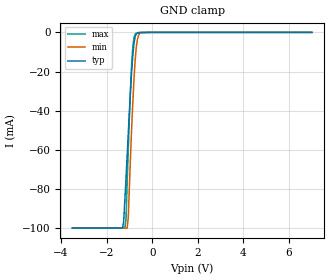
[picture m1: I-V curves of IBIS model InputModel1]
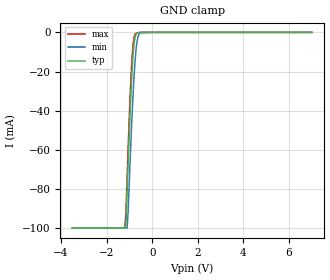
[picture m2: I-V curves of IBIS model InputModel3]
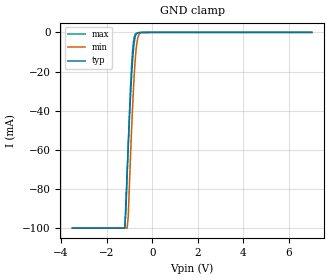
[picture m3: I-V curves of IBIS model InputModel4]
[IBIS Ver]   2.1
[File name]   e_032sa3.ibs   | e_= TSOP, f032sa= abbr chip name, 3= 3.3V Vcc
[File Rev]   2.00
[Date]   26-February-96
[Source]   File generated from lab measurements at Intel Corporation
[Notes]   Rev 2.00   All data from actual measurements performed in a lab.
[Disclaimer] INTEL DEVELOPER'S SOFTWARE LICENSE AGREEMENT
| BY USING THIS SOFTWARE, YOU ARE AGREEING TO BE BOUND
| BY THE TERMS OF THIS AGREEMENT.  DO NOT USE THE SOFTWARE
| UNTIL YOU HAVE CAREFULLY READ AND AGREED TO THE FOLLOWING
| TERMS AND CONDITIONS.  IF YOU DO NOT AGREE TO THE TERMS
| OF THIS AGREEMENT, PROMPTLY RETURN THE SOFTWARE PACKAGE
| AND ANY ACCOMPANYING ITEMS.
| IF YOU USE THIS SOFTWARE, YOU WILL BE BOUND BY THE TERMS
| OF THIS AGREEMENT
| LICENSE: Intel Corporation ("Intel") grants you the non-exclusive right
| to use the enclosed software program ("Software").  You will not use,
| copy, modify, rent, sell or transfer the Software or any portion
| thereof, except as provided in this Agreement.
| System OEM Developers may:
| 1.   Copy the Software for support, backup or archival purposes;
| 2.   Install, use, or distribute Intel owned Software in object code
|   only;
| 3.   Modify and/or use Software source code that Intel directly makes
|   available to you as an OEM Developer;
| 4.   Install, use, modify, distribute, and/or make or have made
|   derivatives ("Derivatives") of Intel owned Software under the
|   terms and conditions in this Agreement, ONLY if you are a System
|   OEM Developer and NOT an end-user.
| RESTRICTIONS:
| YOU WILL NOT:
| 1.   Copy the Software, in whole or in part, except as provided for
|   in this Agreement;
| 2.   Decompile or reverse engineer any Software provided in object
|   code format;
| 3.   Distribute any Software or Derivative code to any end-users,
|   unless approved by Intel in a prior writing.
| TRANSFER: You may transfer the Software to another OEM
| Developer if thereceiving party agrees to the terms of this
| Agreement at the sole risk of any receiving party.
| OWNERSHIP AND COPYRIGHT OF SOFTWARE:
| Title to the Software and all copies thereof remain with Intel
| or its vendors.  The Software iscopyrighted and is protected by
| United States and international copyright laws.  You will not
| remove the copyright notice from the Software.  You agree to
| prevent any unauthorized copying of the Software.
| DERIVATIVE WORK: OEM Developers that make or have made
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[Copyright]   Copyright 1996, Intel Corporation, All Rights Reserved
[Component]   E28F032SA   | 56-lead TSOP package, 28F032SA
[Manufacturer]  Intel   | FlashFile(tm) Memory
|   | operating in 3.3 V Vcc range
|********************Pin and Package Definitions*********************
[Package]
|The following values apply for the Copper leadframe.
|Variable   typ   min   max
R_pkg   48m   41m   54m
L_pkg   4.92nH   4.44nH   5.39nH
C_pkg   0.48pF   0.45pF   0.50pF
|The following values apply for the Alloy-42 leadframe.
|Variable   typ   min   max
|R_pkg   195m   180m   210m
|L_pkg   4.92nH   4.44nH   5.39nH
|C_pkg   0.48pF   0.45pF   0.50pF
|***********************Pin Defintions*************************************
[Pin] signal_name   model_name   R_pin   L_pin   C_pin
  1   3/5#   InputModel1
  2   CE1#   InputModel5
  3   CE2#   InputModel6
  4   A20   InputModel3
  5   A19   InputModel3
  6   A18   InputModel1
  7   A17   InputModel1
  8   A16   InputModel1
  9   VCC   POWER
 10   A15   InputModel1
 11   A14   InputModel3
 12   A13   InputModel1
 13   A12   InputModel1
 14   CE0#   InputModel1
 15   VPP   POWER
 16   RP#   InputModel4
 17   A11   InputModel1
 18   A10   InputModel1
 19   A9   InputModel1
 20   A8   InputModel1
 21   GND   GND
 22   A7   InputModel1
 23   A6   InputModel1
 24   A5   InputModel1
 25   A4   InputModel1
 26   A3   InputModel1
 27   A2   InputModel1
 28   A1   InputModel1
 29   NC   InputModel2
 30   NC   InputModel2
 31   BYTE#   InputModel1
 32   A0   InputModel1
 33   DQ0   InputOutput
 34   DQ8   InputOutput
 35   DQ1   InputOutput
 36   DQ9   InputOutput
 37   VCC   POWER
 38   DQ2   InputOutput
 39   DQ10   InputOutput
 40   DQ3   InputOutput
 41   DQ11   InputOutput
 42   GND   GND
 43   VCC   POWER
 44   DQ4   InputOutput
 45   DQ12   InputOutput
 46   DQ5   InputOutput
 47   DQ13   InputOutput
 48   GND   GND
 49   DQ6   InputOutput
 50   DQ14   InputOutput
 51   DQ7   InputOutput
 52   DQ15   InputOutput
 53   RY/BY#   OpenDrainOutput
 54   OE#   InputModel1
 55   WE#   InputModel4
 56   WP#   InputModel1
|*************************Input Model 2***************************
[Model]   InputModel2
Model_type   Input
|   For NC (Pins 29 & 30)
Vinl = 0.8V
Vinh = 2.0V
| Variable   typ   min   max
C_comp   5.61p   NA   7.6p
[Voltage Range]   3.3V   3.0V   3.6V
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| Models and submodels in the file (8): InputModel1 (Input), InputModel2 (Input), InputModel3 (Input), InputModel4 (Input), InputModel5 (Input), InputModel6 (Input), InputOutput (I/O), OpenDrainOutput (Open_drain)
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|**********************Input Model 1 *******************************
[Model]   InputModel1
Model_type   Input
|   For pin1(3/5#), CE0#, OE#, WP#, BYTE#, A[18:15], A[13:0]
Vinl = 0.8V
Vinh = 2.0V
|Variable   typ   min   max
C_comp   5.61p   NA   7.6p
[Voltage Range]   3.3V   3.0V   3.6V
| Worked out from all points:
|   GND clamp passes 1 mA (typ) near -0.71 V on its own axis
[GND_clamp]
|Voltage I(typ)   I(min)   I(max)
-3.5V     -100mA     -100mA     -100mA
-1.3V     -100mA     -100mA     -100mA
-1.25V    -96.28mA   -100mA     -100mA
-1.2V     -85.5mA    -100mA     -100mA
-1.15V    -74.82mA   -100mA     -95.38mA
-1.1V     -63.19mA   -100mA     -77.19mA
-1.05V    -51.65mA   -94.74mA   -59.72mA
-900mV    -19.67mA   -48.51mA   -16.14mA
-800mV    -5.637mA   -23.94mA   -2.691mA
-700mV    -825.9uA   -7.833mA   -443uA
-500mV    -38.75uA   -204.5uA   -17.62uA
7V        0A         0A         0A
[POWER_clamp]
| Input buffer circuits of this product do not intrinsically
| require a [POWER_clamp] definition.  This zero current
| [POWER_clamp] is provided for compatibility with some ibis
| parsers.
|   Voltage  I(typ)   I(min)   I(max)
-5V       0A         0A         0A
-4.75V    0A         0A         0A
9.75V     0A         0A         0A
10V       0A         0A         0A
|***************************Input Model 3****************************
[Model]   InputModel3
Model_type   Input
|   for A[20], A[19], A[14]
Vinl = 0.8V
Vinh = 2.0V
| Variable   typ   min   max
C_comp   5.61p   NA   7.6p
[Voltage Range]   3.3V   3.0V   3.6V
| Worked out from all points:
|   GND clamp passes 1 mA (typ) near -0.71 V on its own axis
[GND_clamp]
|Voltage I(typ)   I(min)   I(max)
-3.5V     -100mA     -100mA     -100mA
-1.2V     -100mA     -100mA     -100mA
-1.15V    -98.19mA   -100mA     -91.17mA
-1.1V     -81.39mA   -100mA     -73.87mA
-1.05V    -65.32mA   -90.5mA    -57.23mA
-950mV    -35.68mA   -60.49mA   -27.48mA
-900mV    -23.05mA   -46.67mA   -15.71mA
-800mV    -6.001mA   -23.28mA   -2.655mA
-700mV    -807.1uA   -7.759mA   -423.4uA
-600mV    -186uA     -1.489mA   -125.3uA
-500mV    -26.79uA   -201.5uA   -16.26uA
7V        0A         0A         0A
[POWER_clamp]
| Input buffer circuits of this product do not intrinsically
| require a [POWER_clamp] definition.  This zero current
| [POWER_clamp] is provided for compatibility with some ibis
| parsers.
|   Voltage  I(typ)   I(min)   I(max)
-5V       0A         0A         0A
-4.75V    0A         0A         0A
9.75V     0A         0A         0A
10V       0A         0A         0A
|*************************Input Model 4*****************************
[Model]   InputModel4
Model_type   Input
|   for RP#, WE#
Vinl = 0.8V
Vinh = 2.0V
| Variable   typ   min   max
C_comp   5.61p   NA   7.6p
[Voltage Range]   3.3V   3.0V   3.6V
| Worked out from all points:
|   GND clamp passes 1 mA (typ) near -0.70 V on its own axis
[GND_clamp]
|Voltage I(typ)   I(min)   I(max)
-3.5V     -100mA     -100mA     -100mA
-1.2V     -99.74mA   -100mA     -100mA
-1.15V    -85.43mA   -100mA     -90.49mA
-1.1V     -71.41mA   -100mA     -73.44mA
-1.05V    -57.74mA   -94.01mA   -57mA
-950mV    -32.36mA   -62.71mA   -27.54mA
-900mV    -21.46mA   -48.32mA   -15.85mA
-800mV    -6.006mA   -24mA      -2.746mA
-700mV    -869uA     -7.938mA   -449uA
-600mV    -200.2uA   -1.558mA   -133.9uA
-500mV    -40.22uA   -220.4uA   -17.62uA
7V        0A         0A         0A
[POWER_clamp]
| Input buffer circuits of this product do not intrinsically
| require a [POWER_clamp] definition.  This zero current
| [POWER_clamp] is provided for compatibility with some ibis
| parsers.
|   Voltage  I(typ)   I(min)   I(max)
-5V       0A         0A         0A
-4.75V    0A         0A         0A
9.75V     0A         0A         0A
10V       0A         0A         0A
